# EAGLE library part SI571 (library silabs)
ANY-RATE I2C PROGRAMMABLE XO/VCXO Source: si570.pdf
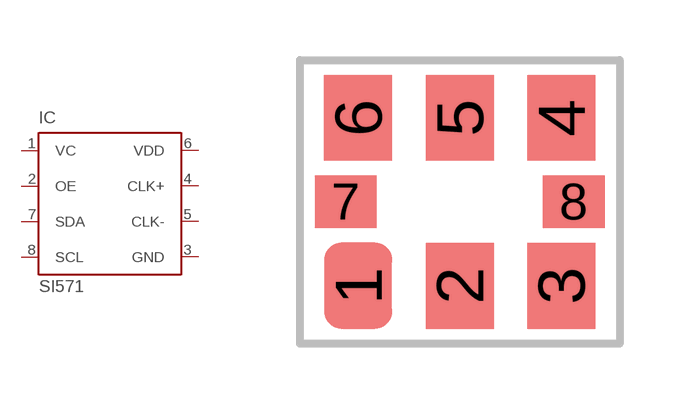
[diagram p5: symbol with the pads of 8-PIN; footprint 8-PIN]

Designator prefix IC

## SI571 (OC_FARNELL: unknown; OC_NEWARK: unknown)  [8-PIN]
1  VC  in
2  OE  in
3  GND  pwr
4  CLK+  out
5  CLK-  out
6  VDD  pwr
7  SDA  in
8  SCL  in

## Footprint 8-PIN (pad centres in mm)
8-Pin PCB Land Pattern Source: si750.pdf
smd 1.7 x 2.15: 1 -2.54,-2.1; 2 0,-2.1; 3 2.54,-2.1; 4 2.54,2.1; 5 0,2.1; 6 -2.54,2.1
smd 1.545 x 1.3: 7 -2.853,0; 8 2.853,0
